(* Logix 5000 AddOnInstructionDefinition export AOI_Bead_Calculate_Limits; software revision 36.00 *)

TYPE DUT_NDSN_spLink_Bead :
STRUCT
   di_rw_NumOfBeads : DINT;
   di_rw_BeadDelay : DINT[8];   // 1/4 mm
   di_rw_BeadDuration : DINT[8];   // 1/4 mm
   di_rw_mode : DINT;   // 1/4 mm
   di_rw_MaxGunTime : DINT;   // microseconds
   di_rw_LineSpeedActivation : DINT;   // 100th m/min
   di_rw_LineSpeedDeactivation : DINT;   // 100th m/min
   di_rw_Interval : DINT;   // 1/4 mm
   di_rw_AdhesiveSavings : DINT;   // 30%-60%
   di_rw_EcoBeadPattern : DINT;   // 0-40, Illegal values: 0,1,11,20,21,30,31,38,39
END_STRUCT
END_TYPE

ADD_ON_INSTRUCTION AOI_Bead_Calculate_Limits   (* revision 1.0 *)
VAR_IN_OUT
   UDDT1 : DUT_NDSN_spLink_Bead; {required}
   di_DelayHi : DINT[8]; {required}
   di_DelayLo : DINT[8]; {required}
   di_DurHi : DINT[8]; {required}
   di_DurLo : DINT[8]; {required}
END_VAR
VAR_INPUT
   b_time_distance_Mode : BOOL; {access Read Only, required}   // Time
END_VAR
VAR_IN_OUT
   i_DotIntervalHi : DINT; {required}
   i_DotIntervalLo : DINT; {required}
END_VAR
VAR
   Max_Hi_Limit : DINT; {access None}
   i_Counter : INT; {access None}
   i_BeadTemp : INT; {access None}
   DotIntHiLimit : INT; {access None}
   DotIntLoLimit : INT; {access None}
END_VAR

ROUTINE Logic   (* structured text *)
   //****************************************************************************************
   //
   //  Subroutine:  Bead_Calculate_Limits
   //
   //  Function:  Calculate the Bead Edit Low and Hi limits for the Delay and Duration.
   //
   //***************************************************************************************
   
   
   //  Init Code
   //
   
   	If (b_time_distance_Mode) Then
   		Max_Hi_Limit := 10000;
   		i_DotIntervalHi := 1000;
   		i_DotIntervalLo := 2;
   	else
   		Max_Hi_Limit := 99999;
   		i_DotIntervalHi := 99999;
   		i_DotIntervalLo := 5;
   	end_if;
   
   	i_BeadTemp := UDDT1.di_rw_NumOfBeads-1;
   
   //
   	FOR i_Counter := 0 TO 7 DO
   
   		If (i_Counter = 0) then			// Special starting Conditions for Lower Delay Limit and High Duration Limit
   			di_DelayLo[i_Counter] := 	0;
   			di_DelayHi[i_Counter] := 	UDDT1.di_rw_BeadDelay[i_Counter + 1] - UDDT1.di_rw_BeadDuration[i_Counter] - 1;
   			di_DurHi[i_Counter] := 		UDDT1.di_rw_BeadDelay[i_Counter + 1] - UDDT1.di_rw_BeadDelay[i_Counter] - 1;
   			di_DurLo[i_Counter] := 		1;			//  ALL Duration Low Limits are set to 1
   		end_if;
   
   		If ((i_Counter < i_BeadTemp) AND (i_Counter > 0)) then
   			di_DelayLo[i_Counter] := 	UDDT1.di_rw_BeadDelay[i_Counter-1] + UDDT1.di_rw_BeadDuration[i_Counter-1] + 1;
   			di_DelayHi[i_Counter] := 	UDDT1.di_rw_BeadDelay[i_Counter + 1] - UDDT1.di_rw_BeadDuration[i_Counter] - 1;
   			di_DurHi[i_Counter] := 		UDDT1.di_rw_BeadDelay[i_Counter + 1] - UDDT1.di_rw_BeadDelay[i_Counter]  - 1;
   			di_DurLo[i_Counter] := 		1;			//  ALL Duration Low Limits are set to 1
   		end_if;
   
   		if ((i_Counter = i_BeadTemp) AND (i_Counter > 0)) then
   			di_DelayLo[i_Counter] := 	UDDT1.di_rw_BeadDelay[i_Counter-1] + UDDT1.di_rw_BeadDuration[i_Counter-1] + 1;
   			di_DelayHi[i_Counter] := 	Max_Hi_Limit;
   			di_DurHi[i_Counter] := 		Max_Hi_Limit;
   			di_DurLo[i_Counter] := 		1;			//  ALL Duration Low Limits are set to 1
   		end_if;
   
   		if ((i_Counter = i_BeadTemp) AND (i_Counter = 0)) then
   			di_DelayLo[i_Counter] := 	0;
   			di_DelayHi[i_Counter] := 	Max_Hi_Limit;
   			di_DurHi[i_Counter] := 		Max_Hi_Limit;
   			di_DurLo[i_Counter] := 		1;			//  ALL Duration Low Limits are set to 1
   		end_if;
   
   		if (i_Counter > i_BeadTemp) then
   			di_DelayLo[i_Counter] := 	0;
   			di_DelayHi[i_Counter] := 	0;
   			di_DurHi[i_Counter] := 		0;
   			di_DurLo[i_Counter] := 		0;
   		end_if;
   
   
   	END_FOR;
END_ROUTINE
END_ADD_ON_INSTRUCTION
